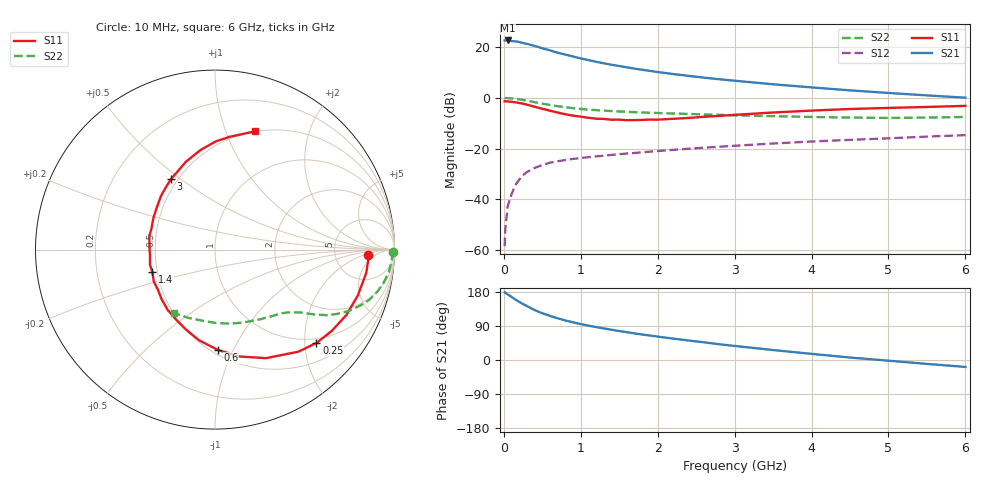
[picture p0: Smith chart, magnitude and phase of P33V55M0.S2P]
! SIEMENS Small Signal Semiconductors
! BFP181
! Si NPN RF Bipolar Junction Transistor in SOT143
! VCE = 3.5 V  IC = 5 mA
! Common Emitter S-Parameters:  March  1996
# GHz  S  MA  R  50
!  f  S11  S21  S12  S22
! GHz  MAG  ANG  MAG  ANG  MAG  ANG  MAG  ANG
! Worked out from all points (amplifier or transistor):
!   36 points, 10 MHz to 6 GHz, reference 50 ohm
!   highest |S21| = 22.6 dB at 50 MHz (marker M1)
!   |S21| within 3 dB of that: start of sweep to 490.3 MHz
!   unconditionally stable (mu >= 1): 1.686 GHz to end of sweep
!   at 250 MHz: K = 0.21, MSG = 26.0 dB, |S12| = -30.5 dB
!   at 1.4 GHz: K = 0.91, MSG = 17.8 dB, |S12| = -22.5 dB
!   at 6 GHz: K = 1.05, MAG = 6.1 dB, |S12| = -14.7 dB
!   lowest NFmin = 1.55 dB at 450 MHz
!   S11 on the Smith chart (normalised r, x): 10 MHz: 12, -3; 250 MHz: 0.89, -2.26; 600 MHz: 0.54, -0.87; 1.4 GHz: 0.47, -0.14; 3 GHz: 0.46, +0.46; 6 GHz: 0.50, +1.27
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0.01  0.8549 -1.9  13.48 178.5  0.0012 91.6  0.992 -0.7
0.02  0.8562 -3.6  13.48 177.5  0.0027 93.5  0.9883 -1.4
0.05  0.8525 -8.8  13.5 173.1  0.0073 90.2  0.9866 -3.9
0.15  0.8177 -26.5  12.96 159.7  0.0191 75.0  0.9571 -11.2
0.2  0.7927 -34.9  12.62 153.4  0.0246 71.5  0.9346 -14.5
0.25  0.7682 -42.6  12.02 147.6  0.03 68.0  0.908 -17.6
0.3  0.7347 -50.7  11.57 142.4  0.0346 64.4  0.8802 -20.1
0.4  0.6684 -64.8  10.56 131.9  0.0416 58.2  0.8214 -24.6
0.5  0.6099 -77.4  9.455 123.4  0.0477 53.2  0.7685 -27.8
0.6  0.5592 -88.3  8.605 116.3  0.0529 50.2  0.7248 -30.3
0.7  0.5131 -99.9  7.737 110.0  0.0564 47.5  0.6853 -32.0
0.8  0.475 -109.7  7.111 104.3  0.0598 45.1  0.6546 -33.4
0.9  0.4459 -119.2  6.52 99.4  0.0628 43.3  0.6261 -34.7
1.1  0.4057 -137.2  5.552 90.5  0.068 41.5  0.5868 -36.6
1.4  0.3706 -160.0  4.492 79.9  0.0753 39.7  0.5491 -39.6
1.8  0.3676 173.3  3.573 67.2  0.0847 38.7  0.5147 -43.5
2.2  0.3865 152.4  2.945 56.4  0.0946 37.4  0.4917 -48.4
3  0.4629 122.0  2.176 37.1  0.1138 33.8  0.4529 -60.1
3.5  0.5148 108.5  1.85 26.3  0.1262 31.2  0.4364 -68.8
4.5  0.6027 89.6  1.405 6.5  0.1489 24.9  0.4089 -89.5
5.5  0.6618 76.6  1.118 -10.3  0.1726 19.3  0.4088 -111.5
6  0.6951 71.4  1.008 -18.3  0.1843 15.7  0.4204 -122.8
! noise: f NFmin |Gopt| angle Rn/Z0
0.45  1.55  0.48  17  0.36
0.9  1.65  0.4  35  0.34
1.8  2  0.18  88  0.34
